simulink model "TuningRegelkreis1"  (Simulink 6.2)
settings: Solver=ode3  StartTime=0.0  StopTime=20  MaxStep=.01  RelTol=1e-3  SampleTimeConstraint=Specified
libraries: simulink_extras x3

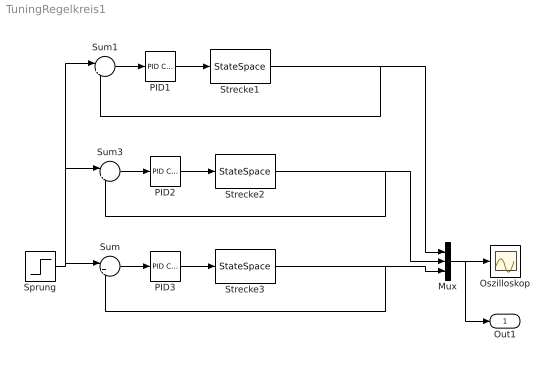
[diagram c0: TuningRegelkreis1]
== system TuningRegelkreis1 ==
  Mux : Mux  Inputs=3
  Oszilloskop : Scope
  PID1 : simulink_extras/Additional Linear/PID Controller  P=26.3  I=0  D=0
  PID2 : simulink_extras/Additional Linear/PID Controller  P=23.7  I=23.7/3.33  D=0
  PID3 : simulink_extras/Additional Linear/PID Controller  P=31.6  I=31.6/2  D=0.5*31.6
  Sprung : Step  Time=2  SampleTime=0
  Strecke1 : StateSpace  A=[-0.404 0.229;0.179 -0.554]  B=[1.189 ;-0.037]  C=[0 0.175]  D=0
  Strecke2 : StateSpace  A=[-0.404 0.229;0.179 -0.554]  B=[1.189 ;-0.037]  C=[0 0.175]  D=0
  Strecke3 : StateSpace  A=[-0.404 0.229;0.179 -0.554]  B=[1.189 ;-0.037]  C=[0 0.175]  D=0
  Sum : Sum  Inputs=|+-
  Sum1 : Sum  Inputs=|+-
  Sum3 : Sum  Inputs=|+-
  Out1 : Outport
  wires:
  PID3/1 -> Strecke3/1
  Sprung/1 -> Sum/1, Sum1/1, Sum3/1
  Sum/1 -> PID3/1
  Strecke3/1 -> Sum/2, Mux/3
  PID1/1 -> Strecke1/1
  Sum1/1 -> PID1/1
  Strecke1/1 -> Sum1/2, Mux/1
  Mux/1 -> Oszilloskop/1, Out1/1
  PID2/1 -> Strecke2/1
  Sum3/1 -> PID2/1
  Strecke2/1 -> Sum3/2, Mux/2
